FUNCTION_BLOCK FB100
TITLE =Set Quick Stop State
//*****************************************************************************
//* maxon motor ag
//* R&D
//* all rights reserved
//*****************************************************************************
//* Summary:  Quick stop device
//*
//* Remarks:
//*
//* Created under: STEP7 REV5.2+SP1
//*****************************************************************************
//* History:
//* 19.05.2004 | INA   first release
//*
//*
//*****************************************************************************
//

AUTHOR:INA
FAMILY:StateMac
NAME:SetQuick
VERSION:00.01


VAR_INPUT

Write : BOOL //A rising edge start the command

  NodeID : BYTE //Adress of the maxon device

END_VAR
VAR_OUTPUT
  Done : BOOL //Data valid flag is TRUE if data were available

  Err : BOOL //Error flag is TRUE if an Error has occured, see ErrNo for more details

  ErrNo : DINT //Contains detailed error information

END_VAR
VAR
  xEdgeMerker : BOOL //Edge Merker

  xEdgeFlag : BOOL //Edge Flag

  xStep : INT
  xQuickStop : WORD  := W#16#2
END_VAR

BEGIN

NETWORK
TITLE = Activate the service function
//

// SDO Write "Set Quick Stop State"

       U    #Write
       FP   #xEdgeFlag                   // recognize a positiv edge of the Read signal
       =    #xEdgeMerker                 // and set the xEdgeMerker for one cycle to true

       L    #xStep
       L    0
       ==I
       U    #xEdgeMerker
       SPB  nstp                         // iStep = 1 -> fnc1

       L    #xStep                       // jump list
       SPL  List
       SPA  rdef
       SPA  fnc1
       SPA  fncE
List  :SPA  rdef

rdef  :NOP  0
       R    #Done                        // reset Done
       R    #Err
       L    0
       T    #xStep                       // iStep = 0
       SPA  end

fnc1  :NOP  0
       CALL FC15
         NodeID:=#NodeID
         Index:=DW#16#00006040
         SubIndex:=DW#16#00000000
         ValueIn:=#xQuickStop
         RET_VAL:=#Done
         Err:=#Err
         ErrNo:=#ErrNo

       L    1
       U    #Err
       SPB  fncE

       SPA  nstp                         // iStep = 1 -> fncE

fncE  :NOP  0
       L    0
       T    #xStep
       SPA  end

nstp  :NOP  0
       L    #xStep
       INC            1
       T    #xStep

end   :NOP  0
END_FUNCTION_BLOCK
